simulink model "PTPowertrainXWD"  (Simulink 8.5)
settings: Solver=ode45  StartTime=0.0  StopTime=inf  RelTol=1e-3
libraries: CarMaker4SL x9, simulink x1
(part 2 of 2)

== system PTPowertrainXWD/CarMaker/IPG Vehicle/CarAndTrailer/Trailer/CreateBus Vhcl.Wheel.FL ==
  In1 : Inport
  Bus Creator3 : BusCreator  Inputs=14
  Demux3 : Demux  Outputs=14
  Out1 : Outport
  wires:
  Demux3/14 -> Bus Creator3/14  "Vhcl Wheel FL Trq_WhlBearing"
  Demux3/13 -> Bus Creator3/13  "Vhcl Wheel FL Trq_T2W"
  Demux3/12 -> Bus Creator3/12  "Vhcl Wheel FL SideSlip"
  Demux3/11 -> Bus Creator3/11  "Vhcl Wheel FL LongSlip"
  Demux3/10 -> Bus Creator3/10  "Vhcl Wheel FL vBelt"
  Demux3/9 -> Bus Creator3/9  "Vhcl Wheel FL Fz"
  Demux3/8 -> Bus Creator3/8  "Vhcl Wheel FL Fy"
  Demux3/7 -> Bus Creator3/7  "Vhcl Wheel FL Fx"
  Demux3/6 -> Bus Creator3/6  "Vhcl Wheel FL r_zxy z"
  Demux3/5 -> Bus Creator3/5  "Vhcl Wheel FL r_zxy y"
  Demux3/4 -> Bus Creator3/4  "Vhcl Wheel FL r_zxy x"
  Demux3/3 -> Bus Creator3/3  "Vhcl Wheel FL t z"
  Demux3/2 -> Bus Creator3/2  "Vhcl Wheel FL t y"
  In1/1 -> Demux3/1
  Bus Creator3/1 -> Out1/1
  Demux3/1 -> Bus Creator3/1  "Vhcl Wheel FL t x"

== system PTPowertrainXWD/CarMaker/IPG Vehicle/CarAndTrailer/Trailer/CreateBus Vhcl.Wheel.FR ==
  In1 : Inport
  Bus Creator3 : BusCreator  Inputs=14
  Demux3 : Demux  Outputs=14
  Out1 : Outport
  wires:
  Demux3/14 -> Bus Creator3/14  "Vhcl Wheel FR Trq_WhlBearing"
  Demux3/13 -> Bus Creator3/13  "Vhcl Wheel FR Trq_T2W"
  Demux3/12 -> Bus Creator3/12  "Vhcl Wheel FR SideSlip"
  Demux3/11 -> Bus Creator3/11  "Vhcl Wheel FR LongSlip"
  Demux3/10 -> Bus Creator3/10  "Vhcl Wheel FR vBelt"
  Demux3/9 -> Bus Creator3/9  "Vhcl Wheel FR Fz"
  Demux3/8 -> Bus Creator3/8  "Vhcl Wheel FR Fy"
  Demux3/7 -> Bus Creator3/7  "Vhcl Wheel FR Fx"
  Demux3/6 -> Bus Creator3/6  "Vhcl Wheel FR r_zxy z"
  Demux3/5 -> Bus Creator3/5  "Vhcl Wheel FR r_zxy y"
  Demux3/4 -> Bus Creator3/4  "Vhcl Wheel FR r_zxy x"
  Demux3/3 -> Bus Creator3/3  "Vhcl Wheel FR t z"
  Demux3/2 -> Bus Creator3/2  "Vhcl Wheel FR t y"
  In1/1 -> Demux3/1
  Bus Creator3/1 -> Out1/1
  Demux3/1 -> Bus Creator3/1  "Vhcl Wheel FR t x"

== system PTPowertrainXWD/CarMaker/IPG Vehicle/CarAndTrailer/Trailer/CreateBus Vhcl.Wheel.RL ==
  In1 : Inport
  Bus Creator3 : BusCreator  Inputs=14
  Demux3 : Demux  Outputs=14
  Out1 : Outport
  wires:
  Demux3/14 -> Bus Creator3/14  "Vhcl Wheel RL Trq_WhlBearing"
  Demux3/13 -> Bus Creator3/13  "Vhcl Wheel RL Trq_T2W"
  Demux3/12 -> Bus Creator3/12  "Vhcl Wheel RL SideSlip"
  Demux3/11 -> Bus Creator3/11  "Vhcl Wheel RL LongSlip"
  Demux3/10 -> Bus Creator3/10  "Vhcl Wheel RL vBelt"
  Demux3/9 -> Bus Creator3/9  "Vhcl Wheel RL Fz"
  Demux3/8 -> Bus Creator3/8  "Vhcl Wheel RL Fy"
  Demux3/7 -> Bus Creator3/7  "Vhcl Wheel RL Fx"
  Demux3/6 -> Bus Creator3/6  "Vhcl Wheel RL r_zxy z"
  Demux3/5 -> Bus Creator3/5  "Vhcl Wheel RL r_zxy y"
  Demux3/4 -> Bus Creator3/4  "Vhcl Wheel RL r_zxy x"
  Demux3/3 -> Bus Creator3/3  "Vhcl Wheel RL t z"
  Demux3/2 -> Bus Creator3/2  "Vhcl Wheel RL t y"
  In1/1 -> Demux3/1
  Bus Creator3/1 -> Out1/1
  Demux3/1 -> Bus Creator3/1  "Vhcl Wheel RL t x"

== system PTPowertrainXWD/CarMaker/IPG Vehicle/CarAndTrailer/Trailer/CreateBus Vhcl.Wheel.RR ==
  In1 : Inport
  Bus Creator3 : BusCreator  Inputs=14
  Demux3 : Demux  Outputs=14
  Out1 : Outport
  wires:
  Demux3/14 -> Bus Creator3/14  "Vhcl Wheel RR Trq_WhlBearing"
  Demux3/13 -> Bus Creator3/13  "Vhcl Wheel RR Trq_T2W"
  Demux3/12 -> Bus Creator3/12  "Vhcl Wheel RR SideSlip"
  Demux3/11 -> Bus Creator3/11  "Vhcl Wheel RR LongSlip"
  Demux3/10 -> Bus Creator3/10  "Vhcl Wheel RR vBelt"
  Demux3/9 -> Bus Creator3/9  "Vhcl Wheel RR Fz"
  Demux3/8 -> Bus Creator3/8  "Vhcl Wheel RR Fy"
  Demux3/7 -> Bus Creator3/7  "Vhcl Wheel RR Fx"
  Demux3/6 -> Bus Creator3/6  "Vhcl Wheel RR r_zxy z"
  Demux3/5 -> Bus Creator3/5  "Vhcl Wheel RR r_zxy y"
  Demux3/4 -> Bus Creator3/4  "Vhcl Wheel RR r_zxy x"
  Demux3/3 -> Bus Creator3/3  "Vhcl Wheel RR t z"
  Demux3/2 -> Bus Creator3/2  "Vhcl Wheel RR t y"
  In1/1 -> Demux3/1
  Bus Creator3/1 -> Out1/1
  Demux3/1 -> Bus Creator3/1  "Vhcl Wheel RR t x"

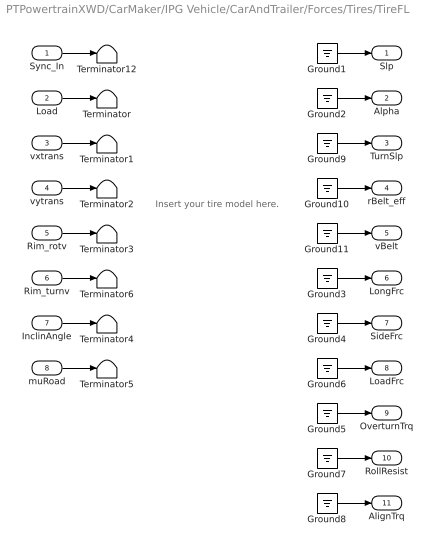
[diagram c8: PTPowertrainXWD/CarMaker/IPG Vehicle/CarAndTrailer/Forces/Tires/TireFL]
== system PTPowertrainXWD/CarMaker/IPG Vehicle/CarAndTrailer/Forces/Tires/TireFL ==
  note: Insert your tire model here.
  Sync_In : Inport
  Load : Inport  Port=2
  vxtrans : Inport  Port=3
  vytrans : Inport  Port=4
  Rim_rotv : Inport  Port=5
  Rim_turnv : Inport  Port=6
  InclinAngle : Inport  Port=7
  muRoad : Inport  Port=8
  Ground{1..11} (11 alike) : Ground
  Terminator{,1..6,12} (8 alike) : Terminator
  Slp : Outport
  Alpha : Outport  Port=2
  TurnSlp : Outport  Port=3
  rBelt_eff : Outport  Port=4
  vBelt : Outport  Port=5
  LongFrc : Outport  Port=6
  SideFrc : Outport  Port=7
  LoadFrc : Outport  Port=8
  OverturnTrq : Outport  Port=9
  RollResist : Outport  Port=10
  AlignTrq : Outport  Port=11
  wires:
  Ground11/1 -> vBelt/1
  Ground10/1 -> rBelt_eff/1
  Ground9/1 -> TurnSlp/1
  Rim_turnv/1 -> Terminator6/1
  Sync_In/1 -> Terminator12/1
  Ground2/1 -> Alpha/1
  Ground3/1 -> LongFrc/1
  Ground4/1 -> SideFrc/1
  Ground5/1 -> OverturnTrq/1
  vxtrans/1 -> Terminator1/1
  vytrans/1 -> Terminator2/1
  Rim_rotv/1 -> Terminator3/1
  InclinAngle/1 -> Terminator4/1
  muRoad/1 -> Terminator5/1
  Load/1 -> Terminator/1
  Ground1/1 -> Slp/1
  Ground6/1 -> LoadFrc/1
  Ground7/1 -> RollResist/1
  Ground8/1 -> AlignTrq/1

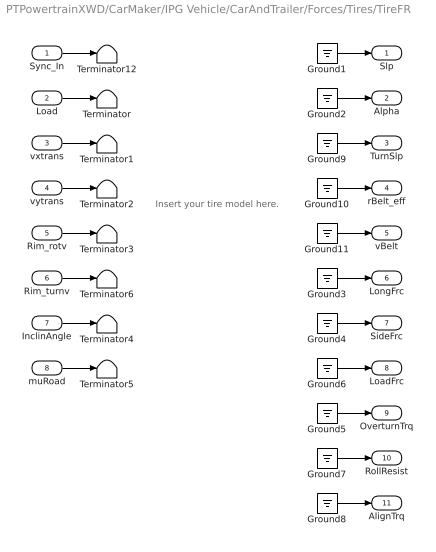
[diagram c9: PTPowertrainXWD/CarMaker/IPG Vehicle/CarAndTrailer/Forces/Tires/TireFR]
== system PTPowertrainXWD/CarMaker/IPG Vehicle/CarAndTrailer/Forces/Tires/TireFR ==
  note: Insert your tire model here.
  Sync_In : Inport
  Load : Inport  Port=2
  vxtrans : Inport  Port=3
  vytrans : Inport  Port=4
  Rim_rotv : Inport  Port=5
  Rim_turnv : Inport  Port=6
  InclinAngle : Inport  Port=7
  muRoad : Inport  Port=8
  Ground{1..11} (11 alike) : Ground
  Terminator{,1..6,12} (8 alike) : Terminator
  Slp : Outport
  Alpha : Outport  Port=2
  TurnSlp : Outport  Port=3
  rBelt_eff : Outport  Port=4
  vBelt : Outport  Port=5
  LongFrc : Outport  Port=6
  SideFrc : Outport  Port=7
  LoadFrc : Outport  Port=8
  OverturnTrq : Outport  Port=9
  RollResist : Outport  Port=10
  AlignTrq : Outport  Port=11
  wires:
  Ground11/1 -> vBelt/1
  Ground10/1 -> rBelt_eff/1
  Ground9/1 -> TurnSlp/1
  Rim_turnv/1 -> Terminator6/1
  Sync_In/1 -> Terminator12/1
  Ground2/1 -> Alpha/1
  Ground3/1 -> LongFrc/1
  Ground4/1 -> SideFrc/1
  Ground5/1 -> OverturnTrq/1
  vxtrans/1 -> Terminator1/1
  vytrans/1 -> Terminator2/1
  Rim_rotv/1 -> Terminator3/1
  InclinAngle/1 -> Terminator4/1
  muRoad/1 -> Terminator5/1
  Load/1 -> Terminator/1
  Ground1/1 -> Slp/1
  Ground6/1 -> LoadFrc/1
  Ground7/1 -> RollResist/1
  Ground8/1 -> AlignTrq/1

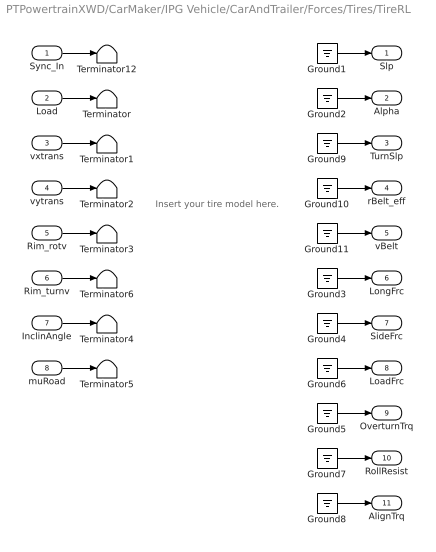
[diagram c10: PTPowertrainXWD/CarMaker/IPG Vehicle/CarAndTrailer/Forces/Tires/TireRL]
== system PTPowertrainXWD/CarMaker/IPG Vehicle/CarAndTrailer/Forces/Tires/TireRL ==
  note: Insert your tire model here.
  Sync_In : Inport
  Load : Inport  Port=2
  vxtrans : Inport  Port=3
  vytrans : Inport  Port=4
  Rim_rotv : Inport  Port=5
  Rim_turnv : Inport  Port=6
  InclinAngle : Inport  Port=7
  muRoad : Inport  Port=8
  Ground{1..11} (11 alike) : Ground
  Terminator{,1..6,12} (8 alike) : Terminator
  Slp : Outport
  Alpha : Outport  Port=2
  TurnSlp : Outport  Port=3
  rBelt_eff : Outport  Port=4
  vBelt : Outport  Port=5
  LongFrc : Outport  Port=6
  SideFrc : Outport  Port=7
  LoadFrc : Outport  Port=8
  OverturnTrq : Outport  Port=9
  RollResist : Outport  Port=10
  AlignTrq : Outport  Port=11
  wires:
  Ground11/1 -> vBelt/1
  Ground10/1 -> rBelt_eff/1
  Ground9/1 -> TurnSlp/1
  Rim_turnv/1 -> Terminator6/1
  Sync_In/1 -> Terminator12/1
  Ground2/1 -> Alpha/1
  Ground3/1 -> LongFrc/1
  Ground4/1 -> SideFrc/1
  Ground5/1 -> OverturnTrq/1
  vxtrans/1 -> Terminator1/1
  vytrans/1 -> Terminator2/1
  Rim_rotv/1 -> Terminator3/1
  InclinAngle/1 -> Terminator4/1
  muRoad/1 -> Terminator5/1
  Load/1 -> Terminator/1
  Ground1/1 -> Slp/1
  Ground6/1 -> LoadFrc/1
  Ground7/1 -> RollResist/1
  Ground8/1 -> AlignTrq/1

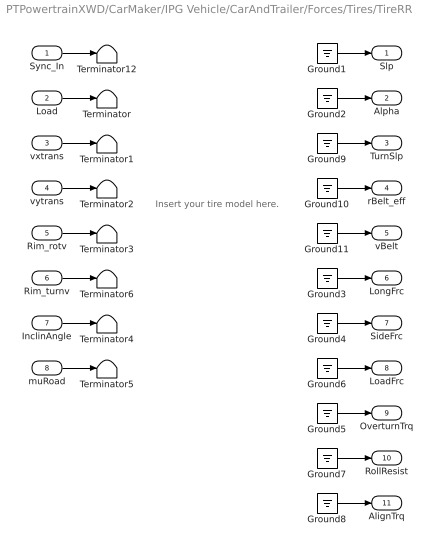
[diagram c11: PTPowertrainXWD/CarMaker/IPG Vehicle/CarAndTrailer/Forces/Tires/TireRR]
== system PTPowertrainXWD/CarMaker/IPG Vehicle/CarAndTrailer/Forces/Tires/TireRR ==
  note: Insert your tire model here.
  Sync_In : Inport
  Load : Inport  Port=2
  vxtrans : Inport  Port=3
  vytrans : Inport  Port=4
  Rim_rotv : Inport  Port=5
  Rim_turnv : Inport  Port=6
  InclinAngle : Inport  Port=7
  muRoad : Inport  Port=8
  Ground{1..11} (11 alike) : Ground
  Terminator{,1..6,12} (8 alike) : Terminator
  Slp : Outport
  Alpha : Outport  Port=2
  TurnSlp : Outport  Port=3
  rBelt_eff : Outport  Port=4
  vBelt : Outport  Port=5
  LongFrc : Outport  Port=6
  SideFrc : Outport  Port=7
  LoadFrc : Outport  Port=8
  OverturnTrq : Outport  Port=9
  RollResist : Outport  Port=10
  AlignTrq : Outport  Port=11
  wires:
  Ground11/1 -> vBelt/1
  Ground10/1 -> rBelt_eff/1
  Ground9/1 -> TurnSlp/1
  Rim_turnv/1 -> Terminator6/1
  Sync_In/1 -> Terminator12/1
  Ground2/1 -> Alpha/1
  Ground3/1 -> LongFrc/1
  Ground4/1 -> SideFrc/1
  Ground5/1 -> OverturnTrq/1
  vxtrans/1 -> Terminator1/1
  vytrans/1 -> Terminator2/1
  Rim_rotv/1 -> Terminator3/1
  InclinAngle/1 -> Terminator4/1
  muRoad/1 -> Terminator5/1
  Load/1 -> Terminator/1
  Ground1/1 -> Slp/1
  Ground6/1 -> LoadFrc/1
  Ground7/1 -> RollResist/1
  Ground8/1 -> AlignTrq/1
